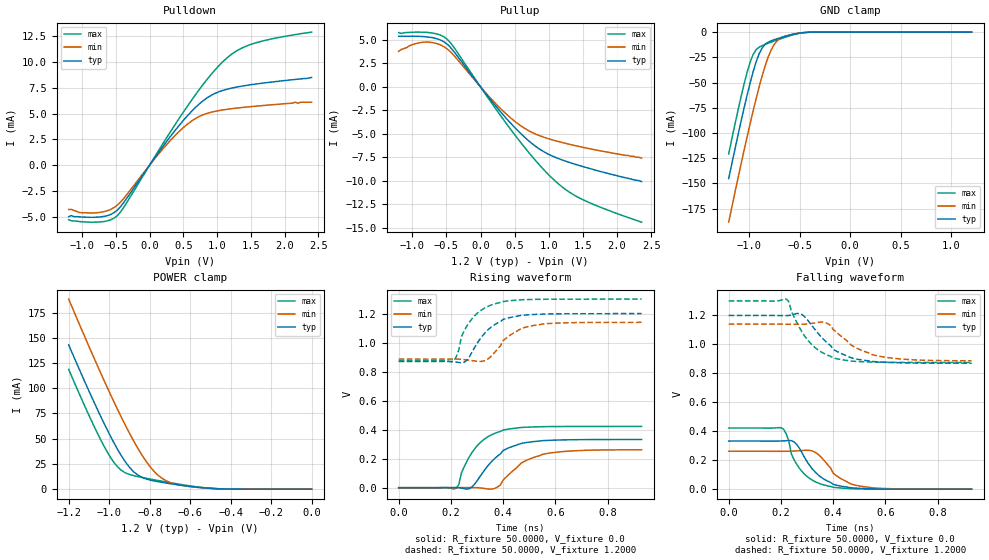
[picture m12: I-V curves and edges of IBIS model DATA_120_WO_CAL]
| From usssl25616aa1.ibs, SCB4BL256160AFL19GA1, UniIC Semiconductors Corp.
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|   Model DATA_120_WO_CAL
[Model]  DATA_120_WO_CAL
Model_type I/O
Polarity   Non-Inverting
Enable   Active-High
Vinl =   0.3800V
Vinh =   0.8200V
Vmeas =  0.6000V
Cref =   5.0000pF
Rref =   50.0000
Vref =   0.6000V
C_comp   1.7430pF   1.7110pF   1.7640pF
[Temperature Range]   25.0000   0.1250k   -40.0000
[Voltage Range]   1.2000V   1.1400V   1.3000V
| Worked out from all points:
|   slope of the pulldown table from 0 to 0.18 V, typ, clamps not added: 108 ohm
|   slope of the pullup table from 0 to 0.18 V, typ, clamps not added: 108 ohm
|   GND clamp passes 1 mA (typ) near -0.50 V on its own axis
|   POWER clamp passes 1 mA (typ) near -0.51 V on its own axis
|   rising waveform, R_fixture 50.0000, V_fixture 0.0: 20-80 % time 103ps typ, 119ps min, 92.6ps max; typ from 0 V to 0.332 V
|   rising waveform, R_fixture 50.0000, V_fixture 1.2000: 20-80 % time 96ps typ, 92.1ps min, 78.1ps max; typ from 0.87 V to 1.2 V
|   falling waveform, R_fixture 50.0000, V_fixture 0.0: 20-80 % time 91.6ps typ, 91.5ps min, 73.1ps max; typ from 0.332 V to 0 V
|   falling waveform, R_fixture 50.0000, V_fixture 1.2000: 20-80 % time 115ps typ, 132ps min, 100ps max; typ from 1.2 V to 0.87 V
[Pulldown]
|Voltage   I(typ)   I(min)   I(max)
-1.2V     -5mA       -4.3mA     -5.3mA
-1V       -5.04mA    -4.63mA    -5.5mA
-760mV    -5.043mA   -4.61mA    -5.523mA
-600mV    -4.846mA   -4.362mA   -5.358mA
-480mV    -4.371mA   -3.891mA   -4.906mA
-360mV    -3.417mA   -3.038mA   -3.855mA
200mV     1.839mA    1.602mA    2.116mA
520mV     4.485mA    3.752mA    5.332mA
840mV     6.469mA    4.992mA    8.219mA
1.2V      7.443mA    5.456mA    10.68mA
1.6V      7.886mA    5.731mA    11.91mA
2.4V      8.5mA      6.1mA      12.9mA
[Pullup]
|Voltage   I(typ)   I(min)   I(max)
-1.2V     5.4mA      3.8mA      5.8mA
-1V       5.41mA     4.51mA     5.83mA
-840mV    5.37mA     4.77mA     5.84mA
-680mV    5.219mA    4.692mA    5.719mA
-520mV    4.73mA     4.215mA    5.263mA
-400mV    3.86mA     3.435mA    4.326mA
120mV     -1.12mA    -992.9uA   -1.272mA
440mV     -3.861mA   -3.297mA   -4.516mA
760mV     -6.076mA   -4.875mA   -7.465mA
1.08V     -7.464mA   -5.705mA   -9.945mA
1.48V     -8.455mA   -6.411mA   -11.96mA
2.36V     -10.1mA    -7.6mA     -14.43mA
[GND_clamp]
|Voltage   I(typ)   I(min)   I(max)
-1.2V     -145.3mA   -188.5mA   -120.8mA
-1.05V    -76.2mA    -118.2mA   -52.43mA
-990mV    -51.2mA    -91.62mA   -30.39mA
-960mV    -39.9mA    -78.82mA   -22.48mA
-900mV    -21.67mA   -54.7mA    -15mA
-870mV    -15.78mA   -43.66mA   -13.45mA
-810mV    -10.04mA   -24.79mA   -11.07mA
-780mV    -8.658mA   -17.59mA   -9.958mA
-720mV    -6.57mA    -8.545mA   -7.793mA
-630mV    -3.906mA   -3.64mA    -4.741mA
-420mV    -215.4uA   -240.5uA   -235uA
1.2V      1.597nA    22.84nA    1.463nA
[POWER_clamp]
|Voltage   I(typ)   I(min)   I(max)
-1.2V     143mA      188.4mA    118.7mA
-1.1V     97.38mA    141.5mA    73.24mA
-1.04V    71.38mA    114.3mA    48.22mA
-1V       55.04mA    96.69mA    33.64mA
-960mV    40mA       79.65mA    22.42mA
-900mV    21.75mA    55.6mA     14.58mA
-860mV    14.17mA    41.05mA    12.52mA
-800mV    9.133mA    22.79mA    10.12mA
-740mV    6.786mA    10.88mA    7.886mA
-660mV    4.332mA    4.436mA    5.101mA
-520mV    1.103mA    1.063mA    1.274mA
0V        1.597nA    6.003nA    2.16nA
[Ramp]
| variable   typ   min   max
dV/dt_r  0.1993/0.1052n   0.1570/0.1198n   0.2534/87.6937p
dV/dt_f  0.1979/0.1159n   0.1521/0.1338n   0.2551/93.0126p
R_load = 50.0000
[Rising Waveform]
R_fixture= 50.0000
V_fixture= 0.0
V_fixture_min= 0.0
V_fixture_max= 0.0
|time   V(typ)   V(min)   V(max)
0s        0V         0V         0V
220ps     1.212mV    171.2uV    -3.906mV
230ps     1.159mV    310uV      20.28mV
250ps     -6.397mV   765.2uV    141mV
290ps     22.9mV     924.5uV    266mV
360ps     188.1mV    -8.825mV   368.4mV
400ps     256.1mV    53.15mV    397.2mV
470ps     305.5mV    170.5mV    414.9mV
550ps     324.1mV    229.5mV    420.4mV
930ps     332.2mV    261.6mV    422.3mV
[Rising Waveform]
R_fixture= 50.0000
V_fixture= 1.2000
V_fixture_min= 1.1400
V_fixture_max= 1.3000
|time   V(typ)   V(min)   V(max)
0s        870mV      885.9mV    874.8mV
210ps     867.6mV    886.4mV    872.9mV
230ps     863.4mV    886mV      948.5mV
240ps     859.7mV    884.2mV    1.04V
280ps     931.8mV    876.2mV    1.163V
340ps     1.085V     885.2mV    1.248V
400ps     1.16V      1.014V     1.283V
470ps     1.188V     1.097V     1.295V
550ps     1.196V     1.128V     1.298V
930ps     1.2V       1.14V      1.3V
[Falling Waveform]
R_fixture= 50.0000
V_fixture= 0.0
V_fixture_min= 0.0
V_fixture_max= 0.0
|time   V(typ)   V(min)   V(max)
0s        332.3mV    261.9mV    422.3mV
210ps     333.4mV    261.5mV    414.3mV
230ps     336.1mV    261.7mV    334.8mV
240ps     335.1mV    262.6mV    242.5mV
270ps     284.7mV    265.5mV    146.3mV
320ps     140.3mV    263.6mV    62.41mV
370ps     63.8mV     188.1mV    26.57mV
420ps     24.55mV    83.48mV    9.531mV
500ps     5.841mV    22.15mV    2.048mV
930ps     3.658uV    23.37uV    748.3nV
[Falling Waveform]
R_fixture= 50.0000
V_fixture= 1.2000
V_fixture_min= 1.1400
V_fixture_max= 1.3000
|time   V(typ)   V(min)   V(max)
0s        1.2V       1.14V      1.3V
220ps     1.199V     1.139V     1.313V
230ps     1.199V     1.139V     1.297V
270ps     1.214V     1.139V     1.119V
300ps     1.173V     1.141V     1.035V
360ps     1.041V     1.154V     941.6mV
400ps     966.4mV    1.103V     906.5mV
470ps     906.6mV    994mV      884.4mV
560ps     880.6mV    924.5mV    876.9mV
930ps     870.1mV    886.5mV    874.8mV
